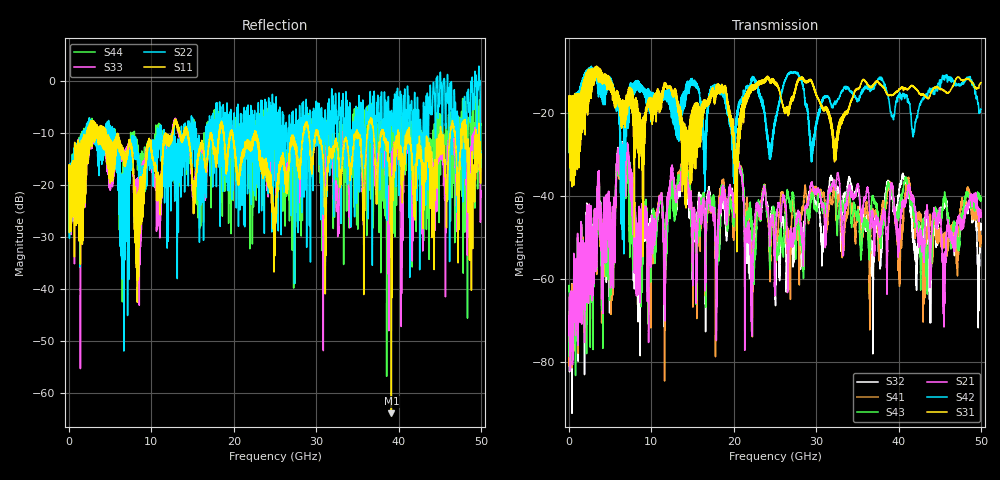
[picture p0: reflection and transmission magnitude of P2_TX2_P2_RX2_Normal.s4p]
!Keysight Technologies,N5225B,MY57041031,A.13.20.10
!Date: Friday, May 31, 2019 11:29:06
!Correction: S11(Full 4 Port(1,2,3,4))
!S12(Full 4 Port(1,2,3,4))
!S13(Full 4 Port(1,2,3,4))
!S14(Full 4 Port(1,2,3,4))
!S21(Full 4 Port(1,2,3,4))
!S22(Full 4 Port(1,2,3,4))
!S23(Full 4 Port(1,2,3,4))
!S24(Full 4 Port(1,2,3,4))
!S31(Full 4 Port(1,2,3,4))
!S32(Full 4 Port(1,2,3,4))
!S33(Full 4 Port(1,2,3,4))
!S34(Full 4 Port(1,2,3,4))
!S41(Full 4 Port(1,2,3,4))
!S42(Full 4 Port(1,2,3,4))
!S43(Full 4 Port(1,2,3,4))
!S44(Full 4 Port(1,2,3,4))
!S4P File: Measurements: <S11,S12,S13,S14>,
!<S21,S22,S23,S24>,
!<S31,S32,S33,S34>,
!<S41,S42,S43,S44>:
# Hz S  dB  R 50.0
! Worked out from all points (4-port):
!   5000 points, 10 MHz to 50 GHz, reference 50 ohm
!   strongest paths, dB at 10 MHz, 12.51 GHz, 25.01 GHz, 37.51 GHz, 50 GHz:
!     S31: -19.4, -14.9, -13.0, -12.4, -12.6
!     S42: -19.6, -15.9, -22.0, -11.6, -18.9
!     S21: -64.4, -32.9, -64.1, -46.1, -44.0
!     S43: -63.0, -38.1, -45.5, -43.9, -40.8
!     S41: -68.0, -35.5, -51.4, -46.9, -50.3
!     S32: -71.4, -35.5, -59.9, -49.3, -46.6
!   lowest |S11| = -63.8 dB at 39.13 GHz (marker M1), VSWR 1.00, Z = 50 + j0.0637 ohm
!   |S11| at or under -10 dB: 4.481 GHz to 11.72 GHz (7.238 GHz wide, 89.4 % of centre); 22.73 GHz to 28.43 GHz (5.701 GHz wide, 22.3 % of centre); 30.26 GHz to 34.82 GHz (4.554 GHz wide, 14 % of centre)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
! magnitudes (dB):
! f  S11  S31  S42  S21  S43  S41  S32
! 10 MHz  -19.1  -19.4  -19.6  -64.4  -63.0  -68.0  -71.4
! 6.43 GHz  -12.8  -17.8  -48.0  -27.6  -27.7  -28.1  -27.3
! 9.74 GHz  -11.0  -18.1  -14.6  -47.7  -49.5  -49.7  -46.5
! 13.9 GHz  -10.2  -32.3  -14.7  -28.8  -29.3  -28.0  -30.1
! 22.18 GHz  -12.1  -14.1  -11.9  -61.4  -48.9  -62.0  -50.7
! 39.13 GHz  -63.8  -15.7  -20.5  -37.2  -38.0  -37.0  -39.4
! 50 GHz  -14.0  -12.6  -18.9  -44.0  -40.8  -50.3  -46.6
